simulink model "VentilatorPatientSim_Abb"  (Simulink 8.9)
settings: Solver=ode3  StartTime=0.0  StopTime=45  FixedStep=0.0001  RelTol=1e-3  EnableMultiTasking=on
undefined symbols (not defined in the file or in its folder): sgn

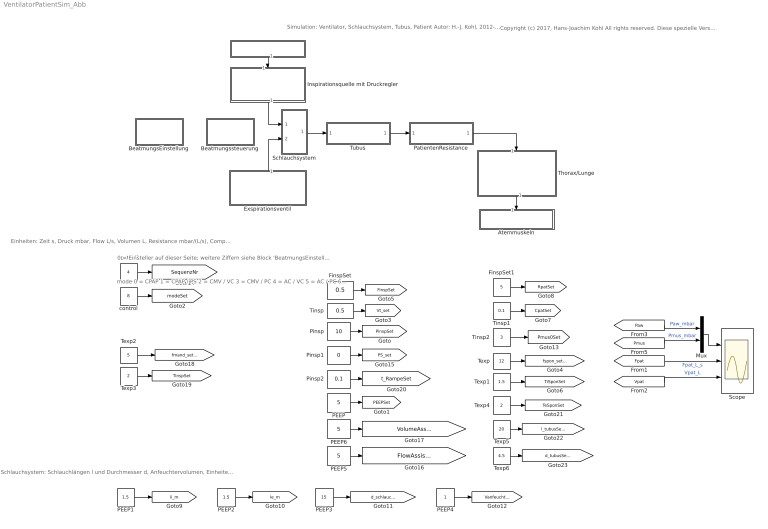
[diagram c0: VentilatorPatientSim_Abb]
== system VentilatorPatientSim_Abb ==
  note: Copyright (c) 2017, Hans-Joachim Kohl All rights reserved. Diese spezielle Version der SW bitte nicht weitergeben (stattdessen gerne die Version mit Namen VentilatorPatientSim, welche die Formulierung einer BSD Lizenz enthält). Sie dient dazu, den Herausgebern des Buches, die Möglichkeit zu geben, die Abb. des Buches nachvollziehen und ggfls. modifizieren zu können. Zusammen mit plotRegulatorModel.m ist sie in der Lage die Abb. des Buch-Beitrages zu reproduzieren, welche nicht beliebig frei verteilt werden dürfen.
  note: Einheiten: Zeit s, Druck mbar, Flow L/s, Volumen L, Resistance mbar/(L/s), Compliance L/mbar
  note: Schlauchsystem: Schlauchlängen l und Durchmesser d, Anfeuchtervolumen, Einheiten siehe Bezeichner
  note: 0 = Einsteller auf dieser Seite; weitere Ziffern siehe Block 'BeatmungsEinstellung'
  note: mode 0 = CPAP 1 = CPAP / PS 2 = CMV / VC 3 = CMV / PC 4 = AC / VC 5 = AC / PC 6 = SIMV / VC 7 = SIMV / PC 8 = CPAP / ATC 9 = CPAP / PPS
  note: Simulation: Ventilator, Schlauchsystem, Tubus, Patient Autor: H.-J. Kohl, 2012-2017. Erstellt für den Beitrag 'Künstliche Beatmung' in 'Medizintechnische Systeme', Springer Vieweg, ISBN 978-3-642-41238-7. Hier werden Signale bereitgestellt, die in plotRegulatorModel.m zu Bildern aufbereitet werden. Vorbereitung: wähle gewünschte SequenzNr und simuliere. Getestet mit Matlab 2014b
  " " : Subsystem
  Atemmuskeln : Subsystem
  BeatmungsEinstellung : Subsystem
  Beatmungssteuerung : Subsystem
  Exspirationsventil : Subsystem
  FinspSet : Constant  Value=0.5
  FinspSet1 : Constant  Value=5
  Inspirationsquelle mit Druckregler : Subsystem
  Mux : Mux  Inputs=2
  PEEP : Constant  Value=5
  PEEP1 : Constant  Value=1.5
  PEEP2 : Constant  Value=1.5
  PEEP3 : Constant  Value=15
  PEEP4 : Constant
  PEEP5 : Constant  Value=5
  PEEP6 : Constant  Value=5
  PatientenResistance : Subsystem
  Pinsp : Constant  Value=10
  Pinsp1 : Constant  Value=0
  Pinsp2 : Constant  Value=0.1
  Schlauchsystem : Subsystem
  Scope : Scope  NumInputPorts=3
  Texp : Constant  Value=12
  Texp1 : Constant  Value=1.5
  Texp2 : Constant  Value=5
  Texp3 : Constant  Value=2
  Texp4 : Constant  Value=2
  Texp5 : Constant  Value=20
  Texp6 : Constant  Value=4.5
  Thorax/Lunge : Subsystem
  Tinsp : Constant  Value=0.5
  Tinsp1 : Constant  Value=0.1
  Tinsp2 : Constant  Value=3
  Tubus : Subsystem
  control : Constant  Value=8  OutDataTypeStr=uint8
  control1 : Constant  Value=4  OutDataTypeStr=uint32  SampleTime=0.0001
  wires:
  Thorax/Lunge/1(Pmus) -> Atemmuskeln/1(" ")
  PatientenResistance/1(" ") -> Thorax/Lunge/1(Palv)
  Pinsp/1 -> [PinspSet]
  PEEP/1 -> [PEEPSet]
  control/1 -> [modeSet]
  Tinsp/1 -> [Vt_set]
  Texp/1 -> [fspon_set_bpm]
  FinspSet/1 -> [FinspSet]
  Texp1/1 -> [TiSponSet]
  Tinsp1/1 -> [CpatSet]
  FinspSet1/1 -> [RpatSet]
  Inspirationsquelle mit Druckregler/1(Finsp) -> Schlauchsystem/1("   ")
  Exspirationsventil/1(" sVentil") -> Schlauchsystem/2(" ")
  Schlauchsystem/1(Paw) -> Tubus/1(Paw)
  PEEP1/1 -> [li_m]
  PEEP2/1 -> [le_m]
  PEEP3/1 -> [d_schlauch_mm]
  PEEP4/1 -> [Vanfeuchter_L]
  Tinsp2/1 -> [Pmus0Set]
  control1/1 -> [SequenzNr]
  Pinsp1/1 -> [PS_set]
  PEEP5/1 -> [FlowAssistSet_mbar__L_s]
  PEEP6/1 -> [VolumeAssistSet_mbar_L]
  Texp2/1 -> [fmand_set_bpm]
  Texp3/1 -> [TinspSet]
  Pinsp2/1 -> [t_RampeSet]
  Texp4/1 -> [TeSponSet]
  Tubus/1(" ") -> PatientenResistance/1(Ptrach)
  Texp5/1 -> [l_tubusSet_cm]
  Texp6/1 -> [d_tubusSet_mm]
  " "/1(" ") -> Inspirationsquelle mit Druckregler/1(" ")
  [Fpat] -> Scope/2  "Fpat_L_s"
  [Vpat] -> Scope/3  "Vpat_L"
  Mux/1 -> Scope/1
  [Paw] -> Mux/1  "Paw_mbar"
  [Pmus] -> Mux/2  "Pmus_mbar"

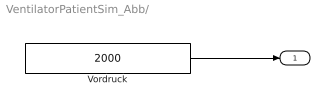
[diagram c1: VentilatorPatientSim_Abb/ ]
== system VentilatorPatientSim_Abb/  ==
  Vordruck : Constant  Value=2000
  " " : Outport
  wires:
  Vordruck/1 -> " "/1

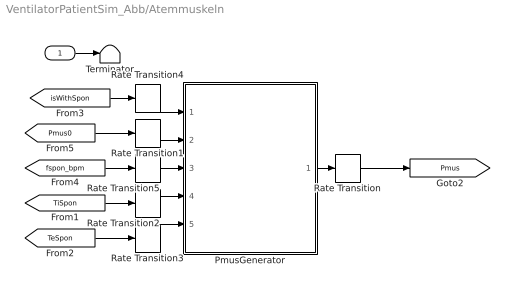
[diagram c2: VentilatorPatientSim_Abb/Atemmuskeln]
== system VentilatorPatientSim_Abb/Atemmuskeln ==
  " " : Inport
  PmusGenerator : Stateflow chart  TreatAsAtomicUnit=on
  Rate Transition{,1..5} (6 alike) : RateTransition  Integrity=off  Deterministic=off
  Terminator : Terminator
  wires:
  " "/1 -> Terminator/1
  PmusGenerator/1(Pmus) -> Rate Transition/1
  [TiSpon] -> Rate Transition2/1
  [TeSpon] -> Rate Transition3/1
  [Pmus0] -> Rate Transition1/1
  Rate Transition/1 -> [Pmus]
  Rate Transition1/1 -> PmusGenerator/2(Pmus0)
  Rate Transition2/1 -> PmusGenerator/4(TiSpon)
  Rate Transition3/1 -> PmusGenerator/5(TeSpon)
  [isWithSpon] -> Rate Transition4/1
  Rate Transition4/1 -> PmusGenerator/1(isWithSpon)
  [fspon_bpm] -> Rate Transition5/1
  Rate Transition5/1 -> PmusGenerator/3(fspon_bpm)

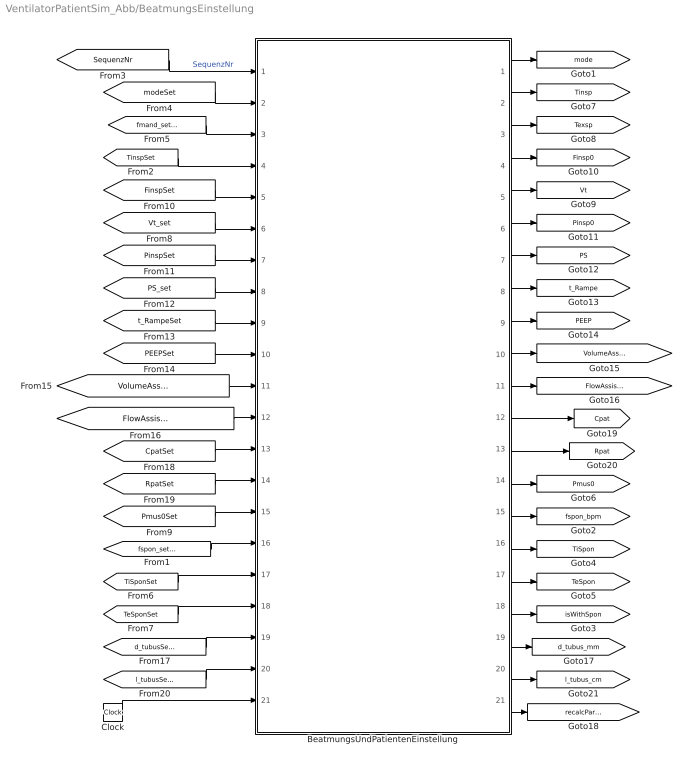
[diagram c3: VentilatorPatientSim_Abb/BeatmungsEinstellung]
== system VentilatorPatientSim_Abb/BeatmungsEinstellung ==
  BeatmungsUndPatientenEinstellung : Stateflow chart  TreatAsAtomicUnit=on
  Clock : Clock
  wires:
  [SequenzNr] -> BeatmungsUndPatientenEinstellung/1(SequenzNr)  "SequenzNr"
  BeatmungsUndPatientenEinstellung/1(mode) -> [mode]
  [modeSet] -> BeatmungsUndPatientenEinstellung/2(modeSet)
  [fmand_set_bpm] -> BeatmungsUndPatientenEinstellung/3(f_set_bpm)
  [TinspSet] -> BeatmungsUndPatientenEinstellung/4(TinspSet)
  BeatmungsUndPatientenEinstellung/18(isWithSpon) -> [isWithSpon]
  BeatmungsUndPatientenEinstellung/16(TiSpon) -> [TiSpon]
  BeatmungsUndPatientenEinstellung/17(TeSpon) -> [TeSpon]
  BeatmungsUndPatientenEinstellung/14(Pmus0) -> [Pmus0]
  BeatmungsUndPatientenEinstellung/2(Tinsp) -> [Tinsp]
  BeatmungsUndPatientenEinstellung/3(Texsp) -> [Texsp]
  [fspon_set_bpm] -> BeatmungsUndPatientenEinstellung/16(fspon_set_bpm)
  [TiSponSet] -> BeatmungsUndPatientenEinstellung/17(TiSponSet)
  [Pmus0Set] -> BeatmungsUndPatientenEinstellung/15(Pmus0Set)
  Clock/1 -> BeatmungsUndPatientenEinstellung/21(time)
  [TeSponSet] -> BeatmungsUndPatientenEinstellung/18(TeSponSet)
  BeatmungsUndPatientenEinstellung/15(fspon_bpm) -> [fspon_bpm]
  [Vt_set] -> BeatmungsUndPatientenEinstellung/6(Vt_set)
  [FinspSet] -> BeatmungsUndPatientenEinstellung/5(FinspSet)
  BeatmungsUndPatientenEinstellung/5(Vt) -> [Vt]
  BeatmungsUndPatientenEinstellung/4(Finsp0) -> [Finsp0]
  [PinspSet] -> BeatmungsUndPatientenEinstellung/7(PinspSet)
  [PS_set] -> BeatmungsUndPatientenEinstellung/8(PS_set)
  [t_RampeSet] -> BeatmungsUndPatientenEinstellung/9(t_RampeSet)
  [PEEPSet] -> BeatmungsUndPatientenEinstellung/10(PEEPSet)
  [VolumeAssistSet_mbar_L] -> BeatmungsUndPatientenEinstellung/11(VolumeAssistSet_mbar_L)
  [FlowAssistSet_mbar__L_s] -> BeatmungsUndPatientenEinstellung/12(FlowAssistSet_mbar__L_s)
  BeatmungsUndPatientenEinstellung/6(Pinsp0) -> [Pinsp0]
  BeatmungsUndPatientenEinstellung/7(PS) -> [PS]
  BeatmungsUndPatientenEinstellung/8(t_Rampe) -> [t_Rampe]
  BeatmungsUndPatientenEinstellung/9(PEEP) -> [PEEP]
  BeatmungsUndPatientenEinstellung/10(VolumeAssist_mbar_L) -> [VolumeAssist_mbar_L]
  BeatmungsUndPatientenEinstellung/11(FlowAssist_mbar__L_s) -> [FlowAssist_mbar__L_s]
  [d_tubusSet_mm] -> BeatmungsUndPatientenEinstellung/19(d_tubusSet_mm)
  BeatmungsUndPatientenEinstellung/19(d_tubus_mm) -> [d_tubus_mm]
  BeatmungsUndPatientenEinstellung/21(recalcParameters) -> [recalcParameters]
  [CpatSet] -> BeatmungsUndPatientenEinstellung/13(CpatSet)
  [RpatSet] -> BeatmungsUndPatientenEinstellung/14(RpatSet)
  [l_tubusSet_cm] -> BeatmungsUndPatientenEinstellung/20(l_tubusSet_cm)
  BeatmungsUndPatientenEinstellung/20(l_tubus_cm) -> [l_tubus_cm]
  BeatmungsUndPatientenEinstellung/12(Cpat) -> [Cpat]
  BeatmungsUndPatientenEinstellung/13(Rpat) -> [Rpat]

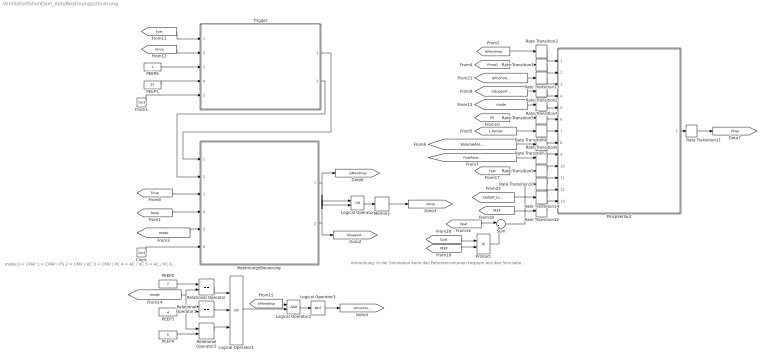
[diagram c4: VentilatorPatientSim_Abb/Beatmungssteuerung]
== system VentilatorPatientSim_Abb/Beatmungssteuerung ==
  note: Anmerkung: in der Simulation kann das Patientenvolumen bequem aus den Simulationsdaten gewonnen werden. In einem Beatmungsgerät ist dafür ein Volumenintegrator erforderlich, der den gemessenen Patientenflow verwendet.
  note: mode 0 = CPAP 1 = CPAP / PS 2 = CMV / VC 3 = CMV / PC 4 = AC / VC 5 = AC / PC 6 = SIMV / VC 7 = SIMV / PC 8 = CPAP / ATC 9 = CPAP / PPS
  BeatmungsSteuerung : Stateflow chart  TreatAsAtomicUnit=on
  Clock : Clock
  Clock1 : Clock
  Logical Operator : Logic  Operator=OR  AllPortsSameDT=off  OutDataTypeStr=boolean
  Logical Operator1 : Logic  Operator=OR  Inputs=3  AllPortsSameDT=off  OutDataTypeStr=boolean
  Logical Operator2 : Logic  AllPortsSameDT=off  OutDataTypeStr=boolean
  Logical Operator3 : Logic  Operator=NOT  AllPortsSameDT=off  OutDataTypeStr=boolean
  Memory : Memory
  PEEP1 : Constant  Value=25
  PEEP2 : Constant  Value=2
  PEEP3 : Constant  Value=4
  PEEP4 : Constant  Value=6
  PEEP6 : Constant  Value=2
  PinspVerlauf : Stateflow chart  TreatAsAtomicUnit=on
  Product : Product
  Rate Transition{1..14} (14 alike) : RateTransition  Integrity=off  Deterministic=off
  Relational Operator : RelationalOperator  Operator===  OutDataTypeStr=boolean
  Relational Operator1 : RelationalOperator  Operator===  OutDataTypeStr=boolean
  Relational Operator2 : RelationalOperator  Operator===  OutDataTypeStr=boolean
  Sum : Sum  Inputs=|+-
  Trigger : Stateflow chart  TreatAsAtomicUnit=on
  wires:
  Trigger/1(isInspTrigger) -> BeatmungsSteuerung/1(isInspTrigger)
  Trigger/2(isExspTrigger) -> BeatmungsSteuerung/2(isExspTrigger)
  [mode] -> BeatmungsSteuerung/5(mode)
  [t_Rampe] -> Rate Transition6/1
  [VolumeAssist_mbar_L] -> Rate Transition7/1
  [FlowAssist_mbar__L_s] -> Rate Transition8/1
  [PS] -> Rate Transition5/1
  BeatmungsSteuerung/1(isMandInsp) -> [isMandInsp], Logical Operator/1
  [Fpat] -> Trigger/1(Fpat)
  PinspVerlauf/1(Pinsp) -> Rate Transition11/1
  [Tinsp] -> BeatmungsSteuerung/3(Tinsp)
  [Texsp] -> BeatmungsSteuerung/4(Texsp)
  [isMandInsp] -> Rate Transition3/1
  BeatmungsSteuerung/2(isSupportedInsp) -> [isSupportedInsp], Logical Operator/2
  [Pinsp0] -> Rate Transition1/1
  [isSupportedInsp] -> Rate Transition2/1
  [mode] -> Rate Transition4/1
  PEEP6/1 -> Trigger/3(FinspTrigger_lpm)
  PEEP1/1 -> Trigger/4(FpercentExspTrigger)
  [isInsp] -> Trigger/2(isInsp)
  Logical Operator/1 -> Memory/1
  [mode] -> Relational Operator/2, Relational Operator1/1, Relational Operator2/1
  Relational Operator/1 -> Logical Operator1/1
  Relational Operator1/1 -> Logical Operator1/2
  [isMandInsp] -> Logical Operator2/1
  Logical Operator1/1 -> Logical Operator2/2
  Logical Operator2/1 -> Logical Operator3/1
  Logical Operator3/1 -> [isPcontrolled]
  PEEP2/1 -> Relational Operator/1
  PEEP3/1 -> Relational Operator1/2
  Clock/1 -> BeatmungsSteuerung/6(time)
  [Fpat] -> Rate Transition9/1
  Rate Transition3/1 -> PinspVerlauf/1(isMandInsp)
  Rate Transition1/1 -> PinspVerlauf/2(PinspSet)
  Rate Transition2/1 -> PinspVerlauf/4(isSuppInsp)
  Rate Transition4/1 -> PinspVerlauf/5(mode)
  Rate Transition5/1 -> PinspVerlauf/6(PS_set)
  Rate Transition6/1 -> PinspVerlauf/7(t_Rampe)
  Rate Transition7/1 -> PinspVerlauf/8(dP_dV)
  Rate Transition8/1 -> PinspVerlauf/9(dP_dFlow)
  Rate Transition9/1 -> PinspVerlauf/10(Fpat)
  Rate Transition10/1 -> PinspVerlauf/11(Vpat)
  Rate Transition11/1 -> [Pinsp]
  [PEEP] -> Rate Transition12/1
  Rate Transition12/1 -> PinspVerlauf/13(Peep)
  Memory/1 -> [isInsp]
  Clock1/1 -> Trigger/5(time)
  [Vpat] -> Sum/1
  Product/1 -> Sum/2
  [PEEP] -> Product/2
  [Cpat] -> Product/1
  Sum/1 -> Rate Transition10/1
  Rate Transition13/1 -> PinspVerlauf/3(isPcontrolled)
  [isPcontrolled] -> Rate Transition13/1
  PEEP4/1 -> Relational Operator2/2
  Relational Operator2/1 -> Logical Operator1/3
  Rate Transition14/1 -> PinspVerlauf/12(DeltaP_tubus)
  [DeltaP_tubus] -> Rate Transition14/1

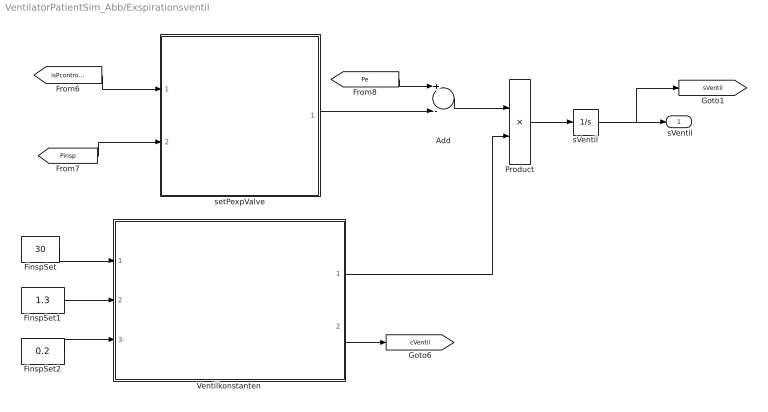
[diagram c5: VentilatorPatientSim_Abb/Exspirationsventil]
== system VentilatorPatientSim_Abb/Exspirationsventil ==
  Add : Sum  Inputs=+-
  FinspSet : Constant  Value=30
  FinspSet1 : Constant  Value=1.3
  FinspSet2 : Constant  Value=0.2
  Product : Product  Inputs=**
  Ventilkonstanten : Stateflow chart  TreatAsAtomicUnit=on
  sVentil : Integrator  LimitOutput=on  UpperSaturationLimit=3  LowerSaturationLimit=0  ContinuousStateAttributes='sVentil'
  setPexpValve : Stateflow chart  TreatAsAtomicUnit=on
  " sVentil" : Outport
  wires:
  [isPcontrolled] -> setPexpValve/1(isPcontrolled)
  [Pinsp] -> setPexpValve/2(Pinsp)
  sVentil/1 -> " sVentil"/1, [sVentil]
  [Pe] -> Add/1
  setPexpValve/1(PexpValve) -> Add/2
  Product/1 -> sVentil/1
  Add/1 -> Product/1
  Ventilkonstanten/1(cVentil_sdot_mm_s__mbar) -> Product/2
  Ventilkonstanten/2(cVentil_flow_L_s__mm___mbar05) -> [cVentil]
  FinspSet/1 -> Ventilkonstanten/1(D_Ventil_mm)
  FinspSet1/1 -> Ventilkonstanten/2(rhoLuft_kg_m3)
  FinspSet2/1 -> Ventilkonstanten/3(tau3mm_s)

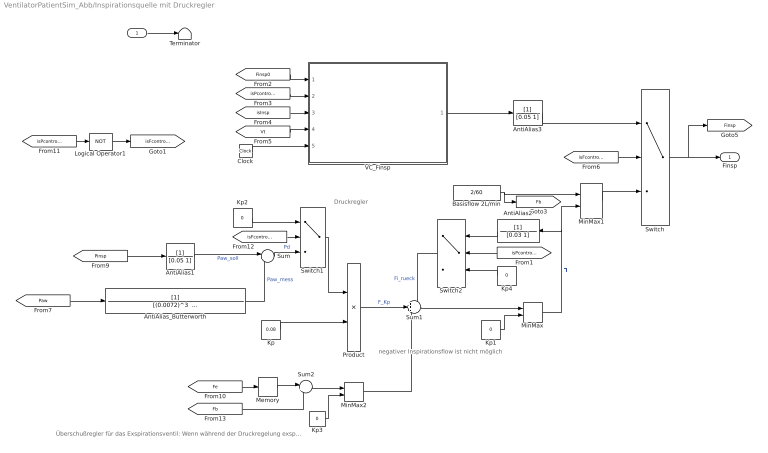
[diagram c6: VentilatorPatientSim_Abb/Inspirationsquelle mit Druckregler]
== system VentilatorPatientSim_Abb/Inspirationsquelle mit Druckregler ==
  note: Druckregler
  note: Überschußregler für das Exspirationsventil: Wenn während der Druckregelung exspiratorisch mehr als der Basisflow fliesst, dann wird der Inspirationsflow bis auf Basisflow zurückgenommen.
  note: negativer Inspirationsflow ist nicht möglich
  " " : Inport
  AntiAlias1 : TransferFcn  Denominator=[0.05 1]
  AntiAlias2 : TransferFcn  Denominator=[0.03 1]
  AntiAlias3 : TransferFcn  Denominator=[0.05 1]
  AntiAlias_Butterworth : TransferFcn  Denominator="[(0.0072)^3   2*(0.0072)^2    2*0.0072   1]"
  Basisflow 2L/min : Constant  Value=2/60
  Clock : Clock
  Kp : Constant  Value=0.08
  Kp{1..4} (4 alike) : Constant  Value=0
  Logical Operator1 : Logic  Operator=NOT  AllPortsSameDT=off  OutDataTypeStr=boolean
  Memory : Memory
  MinMax : MinMax  Function=max  Inputs=2
  MinMax1 : MinMax  Function=max  Inputs=2
  MinMax2 : MinMax  Function=max  Inputs=2
  Product : Product
  Sum : Sum  Inputs=|+-
  Sum1 : Sum  Inputs=++-
  Sum2 : Sum  Inputs=|+-
  Switch : Switch  Criteria=u2 ~= 0  ZeroCross=off
  Switch1 : Switch  Criteria=u2 ~= 0  ZeroCross=off
  Switch2 : Switch  Criteria=u2 ~= 0
  Terminator : Terminator
  VC_Finsp : Stateflow chart  TreatAsAtomicUnit=on
  Finsp : Outport
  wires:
  " "/1 -> Terminator/1
  [Finsp0] -> VC_Finsp/1(Finsp0)
  [isPcontrolled] -> VC_Finsp/2(isPcontrolled)
  [isInsp] -> VC_Finsp/3(isInsp)
  [Vt] -> VC_Finsp/4(Vt)
  Clock/1 -> VC_Finsp/5(time)
  VC_Finsp/1(Finsp) -> AntiAlias3/1
  Switch/1 -> Finsp/1, [Finsp]
  [Paw] -> AntiAlias_Butterworth/1
  [Pinsp] -> AntiAlias1/1
  Kp/1 -> Product/2
  Sum1/1 -> MinMax/1
  MinMax/1 -> MinMax1/2, AntiAlias2/1  "Fi"
  Kp1/1 -> MinMax/2
  Switch2/1 -> Sum1/1  "Fi_rueck"
  Product/1 -> Sum1/2  "F_Kp"
  AntiAlias3/1 -> Switch/1
  MinMax1/1 -> Switch/3
  Basisflow 2L/min/1 -> MinMax1/1, [Fb]
  [isPcontrolled] -> Logical Operator1/1
  Logical Operator1/1 -> [isFcontrolled]
  [isFcontrolled] -> Switch/2
  Kp2/1 -> Switch1/1
  [isFcontrolled] -> Switch1/2
  Sum/1 -> Switch1/3  "Pd"
  Switch1/1 -> Product/1
  AntiAlias1/1 -> Sum/1  "Paw_soll"
  [Fe] -> Memory/1
  [Fb] -> Sum2/2
  Sum2/1 -> MinMax2/1
  Kp3/1 -> MinMax2/2
  MinMax2/1 -> Sum1/3
  Memory/1 -> Sum2/1
  AntiAlias2/1 -> Switch2/1
  [isPcontrolled] -> Switch2/2
  Kp4/1 -> Switch2/3
  AntiAlias_Butterworth/1 -> Sum/2  "Paw_mess"

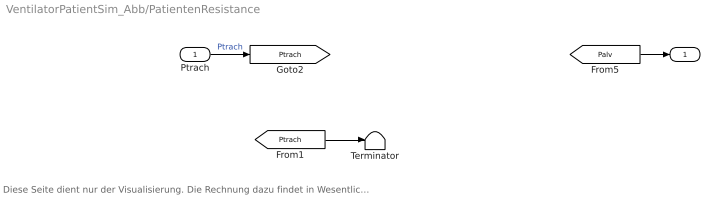
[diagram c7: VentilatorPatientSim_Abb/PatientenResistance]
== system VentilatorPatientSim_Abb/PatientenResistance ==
  note: Diese Seite dient nur der Visualisierung. Die Rechnung dazu findet in Wesentlichen im Block 'Tubus' statt.
  Ptrach : Inport
  Terminator : Terminator
  " " : Outport
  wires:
  [Palv] -> " "/1
  Ptrach/1 -> [Ptrach]  "Ptrach"
  [Ptrach] -> Terminator/1

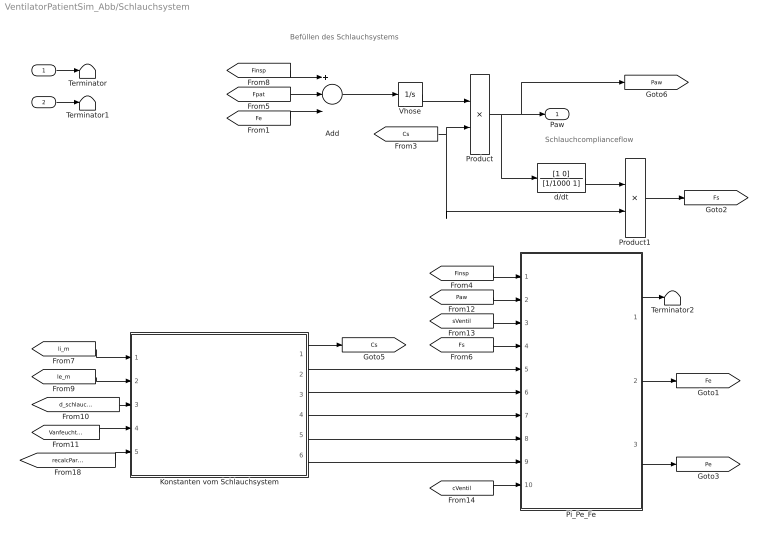
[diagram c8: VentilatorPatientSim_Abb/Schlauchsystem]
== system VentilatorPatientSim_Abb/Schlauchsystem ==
  note: Befüllen des Schlauchsystems
  note: Schlauchcomplianceflow
  "   " : Inport
  " " : Inport  Port=2
  Add : Sum  Inputs=+--
  Konstanten vom Schlauchsystem : Stateflow chart  TreatAsAtomicUnit=on
  Pi_Pe_Fe : Stateflow chart  TreatAsAtomicUnit=on
  Product : Product  Inputs=*/
  Product1 : Product
  Terminator : Terminator
  Terminator1 : Terminator
  Terminator2 : Terminator
  Vhose : Integrator
  d/dt : TransferFcn  Numerator=[1 0]  Denominator=[1/1000 1]
  Paw : Outport
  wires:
  "   "/1 -> Terminator/1
  " "/1 -> Terminator1/1
  [Finsp] -> Add/1
  Vhose/1 -> Product/1
  [Cs] -> Product/2, Product1/2
  Product/1 -> Paw/1, [Paw], d/dt/1
  Product1/1 -> [Fs]
  [Finsp] -> Pi_Pe_Fe/1(Finsp)
  [Fs] -> Pi_Pe_Fe/4(Fs)
  Pi_Pe_Fe/1(Pi) -> Terminator2/1
  Pi_Pe_Fe/2(Fe) -> [Fe]
  Pi_Pe_Fe/3(Pe) -> [Pe]
  Konstanten vom Schlauchsystem/2(i_ie_Cs) -> Pi_Pe_Fe/5(i_ie_Cs)
  [li_m] -> Konstanten vom Schlauchsystem/1(Li_m)
  [le_m] -> Konstanten vom Schlauchsystem/2(Le_m)
  [d_schlauch_mm] -> Konstanten vom Schlauchsystem/3(d_schlauch_mm)
  [Vanfeuchter_L] -> Konstanten vom Schlauchsystem/4(Vanfeuchter_L)
  Konstanten vom Schlauchsystem/1(Cs_L_mbar) -> [Cs]
  [Paw] -> Pi_Pe_Fe/2(Paw)
  Add/1 -> Vhose/1
  d/dt/1 -> Product1/1
  [sVentil] -> Pi_Pe_Fe/3(sVentil_mm)
  [cVentil] -> Pi_Pe_Fe/10(cVentil_l_s__mm___mbar05)
  Konstanten vom Schlauchsystem/3(K1i_mbar__L_s) -> Pi_Pe_Fe/6(K1i)
  Konstanten vom Schlauchsystem/4(K2i_mbar__L2_s2) -> Pi_Pe_Fe/7(K2i)
  Konstanten vom Schlauchsystem/5(K1e_mbar__L_s) -> Pi_Pe_Fe/8(K1e)
  Konstanten vom Schlauchsystem/6(K2e_mbar__L2_s2) -> Pi_Pe_Fe/9(K2e)
  [recalcParameters] -> Konstanten vom Schlauchsystem/5(recalcParameters)
  [Fe] -> Add/3
  [Fpat] -> Add/2

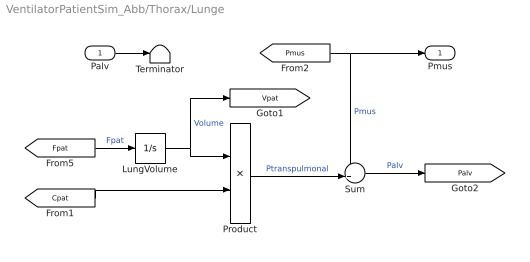
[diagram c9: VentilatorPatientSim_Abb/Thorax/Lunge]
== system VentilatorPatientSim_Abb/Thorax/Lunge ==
  Palv : Inport
  LungVolume : Integrator  ZeroCross=off  ContinuousStateAttributes='LungVolume'
  Product : Product  Inputs=*/
  Sum : Sum  Inputs=++|
  Terminator : Terminator
  Pmus : Outport
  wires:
  [Fpat] -> LungVolume/1  "Fpat"
  LungVolume/1 -> Product/1, [Vpat]  "Volume"
  [Cpat] -> Product/2
  Palv/1 -> Terminator/1
  [Pmus] -> Pmus/1, Sum/1  "Pmus"
  Product/1 -> Sum/2  "Ptranspulmonal"
  Sum/1 -> [Palv]  "Palv"

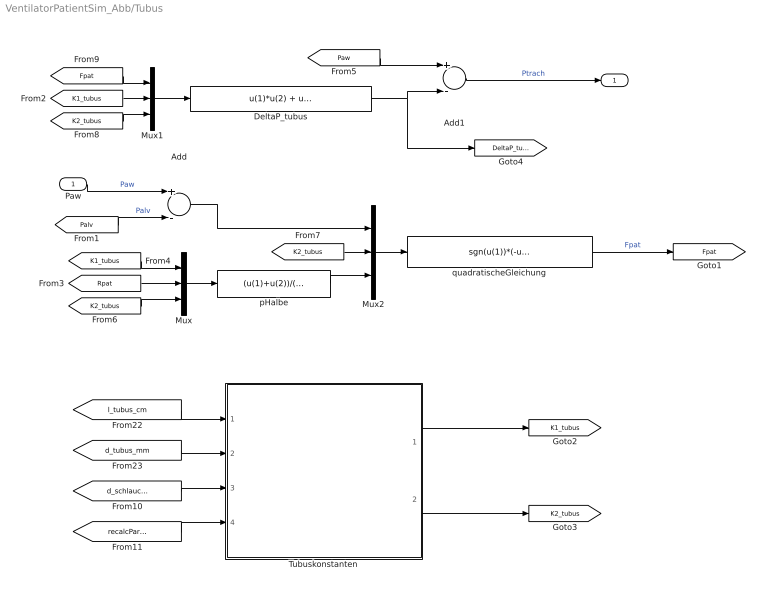
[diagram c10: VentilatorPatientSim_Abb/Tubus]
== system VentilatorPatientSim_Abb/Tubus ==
  Paw : Inport
  Add : Sum  Inputs=+-
  Add1 : Sum  Inputs=+-
  DeltaP_tubus : Fcn  Expr=u(1)*u(2) + u(1)*abs(u(1))*u(3)
  Mux : Mux  Inputs=3
  Mux1 : Mux  Inputs=3
  Mux2 : Mux  Inputs=3
  Tubuskonstanten : Stateflow chart  TreatAsAtomicUnit=on
  pHalbe : Fcn  Expr=(u(1)+u(2))/(2*u(3))
  quadratischeGleichung : Fcn  Expr=sgn(u(1))*(-u(3)+sqrt(u(3)^2+abs(u(1))/u(2)))
  " " : Outport
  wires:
  quadratischeGleichung/1 -> [Fpat]  "Fpat"
  [Palv] -> Add/2  "Palv"
  Paw/1 -> Add/1  "Paw"
  Add/1 -> Mux2/1
  Mux/1 -> pHalbe/1
  [K1_tubus] -> Mux/1
  [Rpat] -> Mux/2
  [K2_tubus] -> Mux/3
  pHalbe/1 -> Mux2/3
  [K2_tubus] -> Mux2/2
  Mux2/1 -> quadratischeGleichung/1
  Mux1/1 -> DeltaP_tubus/1
  [Fpat] -> Mux1/1
  [K1_tubus] -> Mux1/2
  [K2_tubus] -> Mux1/3
  Add1/1 -> " "/1  "Ptrach"
  [Paw] -> Add1/1
  DeltaP_tubus/1 -> Add1/2, [DeltaP_tubus]
  [l_tubus_cm] -> Tubuskonstanten/1(l_tubus_cm)
  [d_tubus_mm] -> Tubuskonstanten/2(d_tubus_mm)
  Tubuskonstanten/1(K1_tubus_mbar__L_s) -> [K1_tubus]
  Tubuskonstanten/2(K2_tubus_mbar__L2_s2) -> [K2_tubus]
  [d_schlauch_mm] -> Tubuskonstanten/3(d_schlauch_mm)
  [recalcParameters] -> Tubuskonstanten/4(recalcParameters)

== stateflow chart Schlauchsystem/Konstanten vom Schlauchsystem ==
  state SchlauchparameterRechnen/
    entry:
    mm_ = 1./1000; cm_ = 1./100; L_ = 1./1000;  mbar_ = 100.; min_ = 60.; s_=1.;
    A = (3.1416/4)*(d_schlauch_mm*mm_)^2;
    V_i = A * Li_m + Vanfeuchter_L * L_;
    V_e = A * Le_m ;
    Cs = (V_i + V_e) / (1013*mbar_);
    i_ie_Cs = V_i / (V_i + V_e);
    K1i = 0.696*mbar_/(L_/s_)*(10/d_schlauch_mm)^4*Li_m;
    Ffix =Li_m^-0.571*(d_schlauch_mm/10)^2.741*250*L_/min_;
    K2i =  (38.8*mbar_/Ffix - K1i) / Ffix;
    K1e =0.696*mbar_/(L_/s_)*(10/d_schlauch_mm)^4*Le_m;
    Ffix =Le_m^-0.571*(d_schlauch_mm/10)^2.741*250*L_/min_;
    K2e = (38.8*mbar_/Ffix - K1e) / Ffix;
    Cs_L_mbar         = Cs / (L_/mbar_);
    K1e_mbar__L_s     = K1e / (mbar_/(L_/s_));
    K2e_mbar__L2_s2 = K2e / (mbar_/(L_/s_)^2);
    K1i_mbar__L_s      = K1i / (mbar_/(L_/s_));
    K2i_mbar__L2_s2  = K2i / (mbar_/(L_/s_)^2);
  (default) -> SchlauchparameterRechnen
  SchlauchparameterRechnen -> SchlauchparameterRechnen : [recalcParameters]

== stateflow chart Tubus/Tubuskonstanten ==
  state Tubus/
    % Rechnungen erfolgen in SI-Basiseinheiten
    entry:
    mm_ = 1./1000; cm_ = 1./100; L_ = 1./1000; mbar_ = 100.; min_ = 60.; s_=1.;
    d_tubus_zu_d_trach = 0.6;
    A_tubus = (3.1416/4)*(d_tubus_mm*mm_)^2;
    A_schlauch = (3.1416/4)*(d_schlauch_mm*mm_)^2;
    A_trachea = (3.1416/4)*(d_tubus_mm*mm_/d_tubus_zu_d_trach)^2;
    rho = 1.21;% kg/m^3
    A2_zu_A1 = A_tubus / A_schlauch;
    Psi = 0.615+0.018*A2_zu_A1+0.1007*A2_zu_A1^2+0.2662*A2_zu_A1^3;
    zeta2 = 1.5*((1-Psi)/Psi)^2;
    K2_s_t = zeta2*(rho/2) / A_tubus^2;
    zeta1 = (1 - A_tubus / A_trachea)^2;
    K2_t_t =  zeta1*(rho/2) / A_trachea^2;
    K1_cyl= 0.696*mbar_/(L_/s_)*(10/d_tubus_mm)^4*(l_tubus_cm*cm_);
    Ffix = (l_tubus_cm*cm_)^-0.571*(d_tubus_mm/10)^2.741*250*L_/min_;
    K2_cyl = (38.8*mbar_/Ffix - K1_cyl) / Ffix;
    K1_tubus_mbar__L_s = K1_cyl / (mbar_/(L_/s_));
    K2_tubus_mbar__L2_s2 = (K2_cyl + K2_s_t + K2_t_t) / (mbar_/(L_/s_)^2);
  Tubus -> Tubus : [recalcParameters]

== stateflow chart Inspirationsquelle
mit
Druckregler/VC_Finsp ==
  state waitForInsp/
  state inspFlowTime/
    entry:
    Finsp = Finsp0;
    tnext = time + TinspFlow;
  state noFlow/
    entry:
    Finsp = 0;
  (default) -> noFlow : {TinspFlow = Vt / Finsp0;}
  waitForInsp -> inspFlowTime : [isInsp]
  noFlow -> waitForInsp : [ ! isInsp && ! isPcontrolled ]
  inspFlowTime -> noFlow : [time >= tnext || isPcontrolled]

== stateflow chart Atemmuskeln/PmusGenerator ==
  state Apnoe/
  state Atmend/
    state insp/
      entry: t=0;
      entry,during:
      Pmus = -Pmus0 * (1-pow(2.7183,-5*t/TiSpon)) / (1-pow(2.7183,-5));
      t = t + 0.001;
    state exp/
      entry: t=0;
      entry,during:
      Pmus = -Pmus0 * (pow(2.7183,-4*t/TeSpon) - pow(2.7183,-4)) / (1-pow(2.7183,-4));
      t = t + 0.001;
    state expPause/
      entry:
      t=0;
      tpause =  60./fspon_bpm - TiSpon - TeSpon;
      entry,during:
      t = t + 0.001;
    (default) -> insp
    insp -> exp : [t > TiSpon]
    expPause -> insp : [t > tpause]
    exp -> expPause : [t > TeSpon]
  (default) -> Apnoe
  Atmend -> Apnoe : [! isWithSpon]
  Apnoe -> Atmend : [isWithSpon]

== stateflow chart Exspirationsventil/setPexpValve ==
  state Pcontrolled/
    entry,during:
    PexpValve = Pinsp;
  state Vcontrolled/
    entry:
    PexpValve = 100;
  Pcontrolled -> Vcontrolled : [ ! isPcontrolled]
  (default) -> Pcontrolled
  Vcontrolled -> Pcontrolled : [isPcontrolled]

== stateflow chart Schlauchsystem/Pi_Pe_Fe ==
  state calc_Pi_Pe_Fe/
    entry, during:
    Fsi = i_ie_Cs * Fs;
    Fse = (Fs - Fsi);
    Pi = Paw + K1i * (Finsp - Fsi/2) + K2i * abs(Finsp - Fsi/2)*(Finsp - Fsi/2);
    fpp = sVentil_mm * cVentil_l_s__mm___mbar05;
    a = 1 + fpp^2 * K2e;
    b = (K1e - K2e * Fse)*fpp;
    c = -Paw + K1e*Fse/2 + K2e*(Fse/2)^2;
    pHalbe = b/(2*a);
    sqrt_Pe = -pHalbe + (pHalbe^2 - c/a)^0.5;
    Pe = sqrt_Pe^2;
    Fe = sqrt_Pe * sVentil_mm * cVentil_l_s__mm___mbar05;
  (default) -> calc_Pi_Pe_Fe

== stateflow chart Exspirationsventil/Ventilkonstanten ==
  state calcVentil/
    entry:
    cVentil_sdot_mm_s__mbar           = (3 / tau3mm_s)/10;                                                       % bei 10mbar Druckdifferenz wird für 3mm die Zeit tau3mm benötigt
    cVentil_flow_L_s__mm___mbar05 = D_Ventil_mm * 3.1416 * sqrt( rhoLuft_kg_m3 / 2) / 100;   % 1/100 = (mm/m) / ((L/cbm)/(mm/m)/(mbar/Pa)^0.5)
  (default) -> calcVentil

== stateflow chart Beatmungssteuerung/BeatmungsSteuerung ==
  state CPAP/
    entry:
    isMandInsp = 0;
    isSupportedInsp = 0;
    state PS/
      entry:
      isSupportedInsp = 1;
      exit:
      isSupportedInsp = 0;
    state noPS/
    (default) -> noPS
    noPS -> PS : [isInspTrigger && mode == 1]
    PS -> noPS : [isExspTrigger]
  state CMV/
    entry:
    isSupportedInsp = 0;
    state exp/
      entry:
      isMandInsp = 0;
      tnext = time + Texsp;
    state insp/
      entry:
      isMandInsp = 1;
      tnext = time + Tinsp;
    (default) -> insp
    insp -> exp : [time >= tnext]
    exp -> insp : [time >= tnext]
  state AC_oder_SIMV/
    entry:
    isSupportedInsp = 0;
    SyncDauer =  min( Texsp-0.5, 5.0);
    tnextSync = time;
    tnextForce = tnextSync + SyncDauer;
    state warteAufTriggerOderForce/
      entry:
      isAC = (mode == 4 || mode == 5);
    state MandStroke/
      entry:
      isMandInsp = 1;
      tnext = time + Tinsp;
      tnextSync = tnextSync + Tinsp + Texsp;
      tnextForce = tnextSync + SyncDauer;
    state verwarteSchutzzeit/
      entry:
      isMandInsp = 0;
      tnext = time + 0.5;
    state erlaubeSupport/
    state PS/
      entry:
      isSupportedInsp = 1;
      exit:
      isSupportedInsp = 0;
    (default) -> warteAufTriggerOderForce
    (junction 165) -> warteAufTriggerOderForce
    (junction 166) -> (junction 165)
    (junction 167) -> (junction 165) : [isAC]
    erlaubeSupport -> (junction 166) : [time >= tnextSync]
    warteAufTriggerOderForce -> MandStroke : [isInspTrigger || time >= tnextForce]
    MandStroke -> verwarteSchutzzeit : [time >= tnext]
    verwarteSchutzzeit -> (junction 167) : [time >= tnext]
    (junction 167) -> erlaubeSupport
    PS -> verwarteSchutzzeit : [isExspTrigger]
    erlaubeSupport -> PS : [isInspTrigger && time < tnextSync]
  (default) -> CPAP
  (junction 192) -> CPAP : [mode == 0 || mode == 1 || mode == 6]
  CPAP -> (junction 192) : [ ! (mode == 0 || mode == 1 || mode == 6)]
  (junction 192) -> CMV : [mode == 2 || mode == 3]
  CMV -> (junction 192) : [ ! (mode == 2 || mode == 3)]
  (junction 192) -> AC_oder_SIMV : [ mode >= 4 && mode <= 7]
  AC_oder_SIMV -> (junction 192) : [ ! (mode >= 4 && mode <= 7)]

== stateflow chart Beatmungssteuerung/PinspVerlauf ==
  state MandInsp/
    entry:
    Pinsp = PinspSet;
    exit:
    Pinsp = Peep;
  state PS/
    entry:
    dP = PS_set * 0.001 / max( t_Rampe, 0.001);
    Pinsp = Peep + dP;
    during:
    Pinsp = min(Pinsp + dP, Peep + PS_set);
    exit:
    Pinsp = Peep;
  state CPAP_ATC/
    entry, during:
    Pinsp = Peep + DeltaP_tubus;
    exit:
    Pinsp = Peep;
  state PPS/
    state PPS_exsp/
      entry: Pinsp = Peep;
      exit: V0 = Vpat;
    state PPS_insp/
      entry, during:
      Pinsp = Peep + max(Vpat - V0,0) * dP_dV + Fpat * dP_dFlow ;
      exit:
      Pinsp = Peep;
    PPS_insp -> PPS_exsp : [Fpat <= 0]
    PPS_exsp -> PPS_insp : [Fpat > 0]
    (default) -> PPS_exsp
  state exsp/
    Pinsp = Peep;
  (junction 228) -> MandInsp : [isMandInsp && isPcontrolled]
  MandInsp -> (junction 228) : [ ! (isMandInsp && isPcontrolled)]
  (junction 228) -> PS : [isSuppInsp]
  (default) -> (junction 228)
  PS -> (junction 228) : [ ! isSuppInsp]
  (junction 228) -> exsp
  (junction 228) -> CPAP_ATC : [mode == 8]
  exsp -> (junction 228) : [(isMandInsp && isPcontrolled) || isSuppInsp || mode == 8 || mode == 9]
  CPAP_ATC -> (junction 228) : [ ! (mode == 8)]
  PPS -> (junction 228) : [ ! (mode == 9)]
  (junction 228) -> PPS : [mode == 9]

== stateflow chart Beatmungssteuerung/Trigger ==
  state insp/
    entry:
    FiMax = Fpat;
    during:
    FiMax = max(Fpat, FiMax);
  state exsp_insp_is_triggered/
    entry:
    isInspTrigger = 1;
    tnext = time + 0.01;
  state switchToInsp/
    exit:
    isInspTrigger = 0;
  state exsp/
  state insp_exsp_is_triggered/
    entry:
    isExspTrigger = 1;
    tnext = time + 0.01;
  state switchToExsp/
    exit:
    isExspTrigger = 0;
  state WarteAufExspFlow/
  switchToInsp -> insp : [isInsp]
  exsp_insp_is_triggered -> switchToInsp : [time >= tnext]
  switchToInsp -> (junction 260)
  exsp -> exsp_insp_is_triggered : [Fpat > FinspTrigger_lpm/60. && ! isInsp]
  (junction 258) -> insp
  exsp -> (junction 258) : [isInsp]
  insp -> insp_exsp_is_triggered : [Fpat < FiMax * FpercentExspTrigger/100. && isInsp]
  insp -> (junction 259) : [ ! isInsp]
  (junction 259) -> (junction 260)
  (junction 260) -> exsp
  (default) -> exsp : {FiMax=0;  isInspTrigger = 0;  isExspTrigger = 0;}
  switchToExsp -> WarteAufExspFlow : [! isInsp]
  insp_exsp_is_triggered -> switchToExsp : [time >= tnext]
  WarteAufExspFlow -> exsp : [Fpat < 0]

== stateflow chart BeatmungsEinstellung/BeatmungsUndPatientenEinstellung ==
  state SchlauchFuellen/
    entry:
    tnext = time + 1.5;
    mode = 0;
    isWithSpon = 0;
    Tinsp = TinspSet;
    Texsp = 60.0/f_set_bpm - Tinsp;
    fspon_bpm = fspon_set_bpm;
    TiSpon = TiSponSet;
    TeSpon = TeSponSet;
    Pmus0 = Pmus0Set;
    Finsp0 = FinspSet;
    Vt = Vt_set;
    PS = PS_set;
    Pinsp0 = PinspSet;
    t_Rampe = t_RampeSet;
    PEEP = PEEPSet;
    VolumeAssist_mbar_L = VolumeAssistSet_mbar_L;
    FlowAssist_mbar__L_s = FlowAssistSet_mbar__L_s;
    Cpat = CpatSet;
    Rpat = RpatSet;
    d_tubus_mm = d_tubusSet_mm;
    l_tubus_cm = l_tubusSet_cm;
    recalcParameters = 0;
  state SetByParameters/
    entry:
    mode = modeSet;
    isWithSpon = 1;
  state CPAP/
    entry:
    tnext = time + 12;
    mode = 0;
    isWithSpon = 1;
    PEEP = 5;
    Cpat = 0.1;
    Rpat = 5;
    TiSpon = 1.3;
    TeSpon = 2.;
    fspon_bpm = 15;
    Pmus0 = 3;
    d_tubus_mm = 4.5;
    l_tubus_cm = 20;
    recalcParameters = 1;
  state CMV_VC/
    entry:
    tnext = time + 19;
    mode = 2;
    isWithSpon = 0;
    Tinsp = 2;
    f_bpm = 12;
    Texsp = 60.0/f_bpm - Tinsp;
    Finsp0 = 0.5;
    Vt = 0.5;
    PEEP = 5;
    Cpat = 0.1;
    Rpat = 5;
    d_tubus_mm = 8;
    l_tubus_cm = 20;
    recalcParameters = 1;
  state VC_versus_PC/
    entry:
    tnext = time + 19;
    mode = 2;
    isWithSpon = 0;
    Tinsp = 2;
    f_bpm = 12;
    Texsp = 60.0/f_bpm - Tinsp;
    Finsp0 = 0.5;
    Vt = 0.5;
    PEEP = 5;
    Cpat = 0.1;
    Rpat = 5;
    d_tubus_mm = 30; % kein Tubus
    l_tubus_cm = 0;
    recalcParameters = 1;
  state simuliere3/
    entry:
    recalcParameters = 0;
  state simuliere1/
    entry:
    recalcParameters = 0;
  state simuliere4/
    entry:
    recalcParameters = 0;
  state AC_PC/
    entry:
    mode = 5;
    isWithSpon = 1;
    Pinsp0 = 10;
    TiSpon = 0.4;
    TeSpon = 0.4;
    fspon_bpm = 15;
    Pmus0 = 1.5;
  state CPAP_PS/
    entry:
    tnext = time + 8;
    mode = 1;
    PS = 5;
  state PC/
    entry:
    mode = 3;
    Pinsp0 = 10;
  state SIMV_PC/
    entry:
    mode = 7;
    isWithSpon = 1;
    Tinsp = 2;
    f_bpm = 6;
    Texsp = 60.0/f_bpm - Tinsp;
    Pinsp0 = 10;
    PEEP = 5;
    PS = 0;
    Cpat = 0.1;
    Rpat = 5;
    TiSpon = 1.5;
    TeSpon = 2.0;
    fspon_bpm = 15;
    Pmus0 = 3;
    d_tubus_mm = 8;
    l_tubus_cm = 20;
    recalcParameters = 1;
  state CPAP_ATC/
    entry:
    tnext = time + 12;
    mode = 8;
  state simuliere2/
    entry:
    recalcParameters = 0;
  state CPAP_PPS/
    entry:
    tnext = time + 12;
    mode = 9;
  (default) -> SchlauchFuellen
  SchlauchFuellen -> (junction 336) : [time >= tnext]
  (junction 336) -> SetByParameters
  (junction 336) -> (junction 339) : [SequenzNr > 0]
  (junction 337) -> (junction 338)
  (junction 339) -> (junction 337) : [SequenzNr == 4]
  (junction 338) -> VC_versus_PC
  (junction 339) -> CMV_VC : [SequenzNr == 1]
  (junction 339) -> CPAP : [SequenzNr == 3]
  (junction 339) -> (junction 340)
  CPAP -> simuliere3
  VC_versus_PC -> simuliere4
  CMV_VC -> simuliere1
  simuliere3 -> CPAP_PS : [time > tnext]
  simuliere1 -> AC_PC : [time > tnext]
  simuliere4 -> PC : [time > tnext]
  CPAP_PS -> CPAP_ATC : [time > tnext]
  (junction 340) -> SIMV_PC : [ SequenzNr == 2]
  CPAP_ATC -> CPAP_PPS : [time > tnext]
  SIMV_PC -> simuliere2
